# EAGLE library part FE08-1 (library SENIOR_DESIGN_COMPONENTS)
FEMALE HEADER
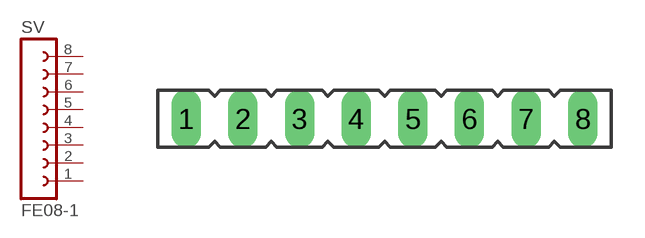
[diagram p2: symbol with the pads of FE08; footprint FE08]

Designator prefix SV

## FE08-1 (OC_FARNELL: unknown; OC_NEWARK: unknown)  [FE08]
1  1  pas
2  2  pas
3  3  pas
4  4  pas
5  5  pas
6  6  pas
7  7  pas
8  8  pas

## Footprint FE08 (pad centres in mm)
FEMALE HEADER
drill 0.813 long: 1 -8.89,0; 2 -6.35,0; 3 -3.81,0; 4 -1.27,0; 5 1.27,0; 6 3.81,0; 7 6.35,0; 8 8.89,0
